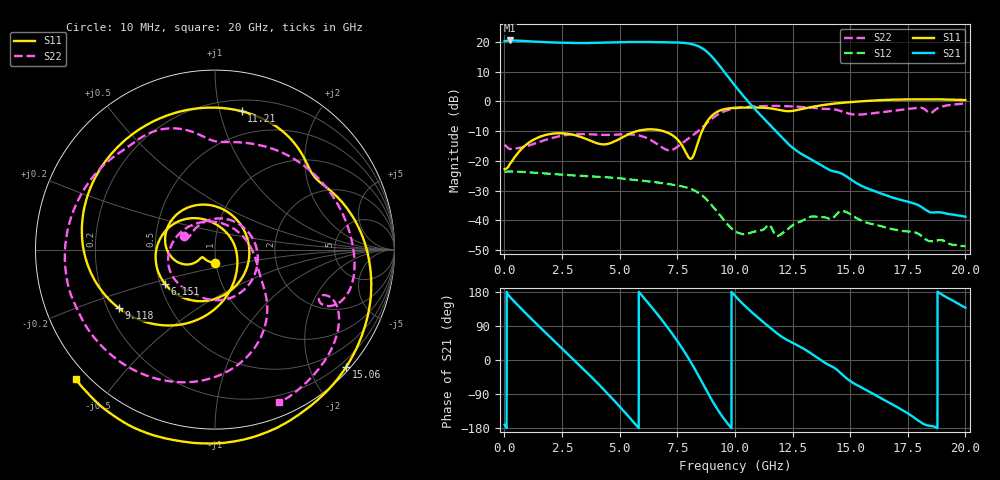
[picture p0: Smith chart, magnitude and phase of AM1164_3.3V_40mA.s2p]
!Agilent Technologies,E8364B,MY43040894,A.07.50.67
!Agilent E8364B: A.07.50.67
!Date: Wednesday, June 12, 2019 11:14:06
!Correction: S11(Full 2 Port(1,2))
!S21(Full 2 Port(1,2))
!S12(Full 2 Port(1,2))
!S22(Full 2 Port(1,2))
!S2P File: Measurements: S11, S21, S12, S22:
# Hz S  dB  R 50
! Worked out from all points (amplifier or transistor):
!   6401 points, 10 MHz to 20 GHz, reference 50 ohm
!   highest |S21| = 20.5 dB at 231.8 MHz (marker M1)
!   |S21| within 3 dB of that: start of sweep to 8.654 GHz
!   unconditionally stable (mu >= 1): start of sweep to 15.35 GHz
!   at 3.34 GHz: K = 1.13, MAG = 20.1 dB, |S12| = -25.0 dB
!   at 10.01 GHz: K = 6.74, MAG = 13.2 dB, |S12| = -43.7 dB
!   at 20 GHz: K = -206.53, MSG = 4.9 dB, |S12| = -48.7 dB
!   S11 on the Smith chart (normalised r, x): 10 MHz: 0.99, -0.14; 6.151 GHz: 0.53, -0.23; 9.118 GHz: 0.25, -0.26; 11.21 GHz: 0.29, +1.17; 15.06 GHz: 0.08, -2.61; 20 GHz: -0.03, -0.39
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1e7  -22.82 -88.9  20.31 -171.0  -23.68 10.0  -14.58 155.9
2.317641e8  -21.14 -149.3  20.54 167.2  -23.54 -10.3  -15.96 151.0
9.376609e8  -14.59 -153.6  20.32 122.7  -23.76 -48.0  -15.09 81.2
1.615447e9  -11.67 -176.5  20.04 82.3  -24.12 -82.3  -13.36 21.6
2.539984e9  -10.70 143.5  19.74 28.3  -24.65 -128.3  -11.45 -40.8
3.342708e9  -12.00 97.9  19.67 -18.8  -25.02 -169.0  -10.94 -80.0
4.104827e9  -14.24 33.1  19.78 -65.0  -25.34 150.4  -11.17 -106.8
4.71702e9  -13.66 -34.2  19.91 -104.1  -25.67 116.5  -11.20 -123.2
5.513497e9  -10.59 -103.4  20.03 -157.7  -26.28 70.8  -11.10 -150.7
6.150678e9  -9.43 -145.1  20.03 157.0  -26.81 33.5  -12.21 174.7
6.675416e9  -9.59 -175.3  19.98 117.9  -27.30 1.1  -14.59 132.3
7.30635e9  -11.44 146.9  19.91 67.2  -27.99 -41.1  -16.18 50.7
7.956025e9  -18.39 67.0  19.57 7.7  -29.07 -91.0  -12.61 -14.1
8.240258e9  -17.47 -21.5  19.09 -21.6  -29.95 -115.9  -11.00 -28.2
8.561972e9  -10.24 -85.2  18.00 -57.1  -31.53 -145.4  -8.92 -39.4
9.117944e9  -4.04 -148.9  14.10 -117.8  -36.06 167.6  -5.11 -63.0
1.0005e10  -2.13 143.5  5.34 169.5  -43.67 129.1  -2.33 -105.2
1.120752e10  -2.10 79.1  -5.36 101.3  -43.21 93.8  -1.56 -148.4
1.333771e10  -1.83 8.6  -19.58 15.9  -38.72 10.4  -2.08 146.9
1.505872e10  -0.17 -41.9  -26.41 -57.8  -38.18 -76.4  -4.27 92.2
1.667042e10  0.57 -79.5  -31.92 -112.1  -42.66 -126.2  -3.32 42.8
2e10  0.49 -136.9  -38.78 138.2  -48.68 131.5  -0.69 -67.1
